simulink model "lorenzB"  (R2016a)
settings: Solver=ode45  StartTime=0.0  StopTime=50.0  MaxStep=1e-2  RelTol=1e-3
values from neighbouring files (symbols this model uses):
  phi = block.InputPort(1).Data    [sfun_pendelstangeanim.m]
undefined symbols (not defined in the file or in its folder): psi, theta, xlims, ylims, zlims
libraries: simulink x3

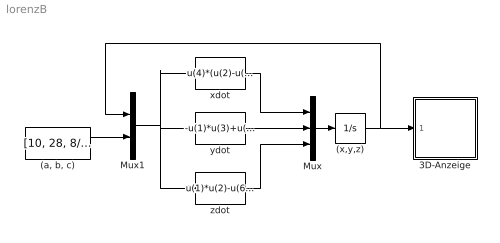
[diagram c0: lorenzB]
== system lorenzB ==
  "(a, b, c)" : Constant  Value=[10, 28, 8/3]
  (x,y,z) : Integrator  InitialCondition=[15 15 15]
  3D-Anzeige : Subsystem
  Mux : Mux  Inputs=3
  Mux1 : Mux  Inputs=2
  xdot : Fcn  Expr=u(4)*(u(2)-u(1))
  ydot : Fcn  Expr=-u(1)*u(3)+u(5)*u(1)-u(2)
  zdot : Fcn  Expr=u(1)*u(2)-u(6)*u(3)
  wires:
  Mux/1 -> (x,y,z)/1
  xdot/1 -> Mux/1
  ydot/1 -> Mux/2
  zdot/1 -> Mux/3
  (x,y,z)/1 -> Mux1/1, 3D-Anzeige/1(In)
  "(a, b, c)"/1 -> Mux1/2
  Mux1/1 -> ydot/1, xdot/1, zdot/1

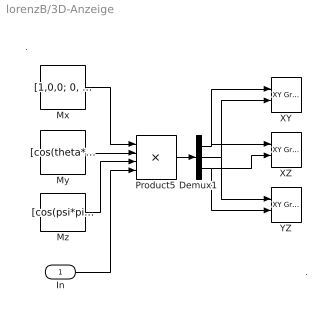
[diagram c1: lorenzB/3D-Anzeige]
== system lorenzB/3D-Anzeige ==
  note: .
  note: .
  In : Inport
  Demux1 : Demux  Outputs=3
  Mx : Constant  Value=[1,0,0; 0, cos(phi*pi/180), -sin(phi*pi/180); 0, sin(phi*pi/180), cos(phi*pi/180)]
  My : Constant  Value=[cos(theta*pi/180),0, sin(theta*pi/180); 0,1,0; -sin(theta*pi/180),0,cos(theta*pi/180)]
  Mz : Constant  Value=[cos(psi*pi/180),-sin(psi*pi/180), 0; sin(psi*pi/180), cos(psi*pi/180), 0; 0,0,1]
  Product5 : Product  Inputs=4  Multiplication=Matrix(*)
  XY : simulink/Sinks/XY Graph  SystemSampleTime=-1  xmin=xlims(1)  xmax=xlims(2)  ymin=ylims(1)  ymax=ylims(2)  st=-1
  XZ : simulink/Sinks/XY Graph  SystemSampleTime=-1  xmin=xlims(1)  xmax=xlims(2)  ymin=zlims(1)  ymax=zlims(2)  st=-1
  YZ : simulink/Sinks/XY Graph  SystemSampleTime=-1  xmin=ylims(1)  xmax=ylims(2)  ymin=zlims(1)  ymax=zlims(2)  st=-1
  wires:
  Demux1/1 -> XZ/1, XY/1
  In/1 -> Product5/4
  Mx/1 -> Product5/1
  My/1 -> Product5/2
  Mz/1 -> Product5/3
  Product5/1 -> Demux1/1
  Demux1/3 -> YZ/2, XZ/2
  Demux1/2 -> YZ/1, XY/2
